| IBIS file stm32f373_378_383_lqfp64.ibs
[IBIS ver] 4.2
[File name] stm32f373_378_383_lqfp64.ibs
[File Rev] 1.0
[Date]  29-09-2025
[Source] Data Created at STMicroelectronics
[Notes]  File originated from ELDO simulations.
[Disclaimer]  This information is for modeling purpose only and is
   not guaranted. The information is subject to change without
   notice.
[Copyright] Copyright 2025 STMicroelectronics Inc.
|   Component stm32f373_378_383_lqfp64
[Component] stm32f373_378_383_lqfp64
[Manufacturer] STMicroelectronics
[Package]
| variable   typ   min   max
R_pkg  0  NA  NA
L_pkg  0  NA  NA
C_pkg  0  NA  NA
[Pin]   signal_name   model_name R_pin  L_pin C_pin
1 VBAT POWER 0.06898 4.22E-09 1.2E-13
2 PC13 io8p_sudq_tc_v33 0.063756122 3.67878E-09 9.34694E-14
3 PC14-OSC32IN io8p_sudq_tc_v33 0.059335918 3.22082E-09 7.10204E-14
4 PC15-OSC32OUT io8p_sudq_tc_v33 0.055719388 2.84612E-09 5.26531E-14
5 PF0/OSC_IN io8p_wsudqh_i2c_ft 0.052906531 2.55469E-09 3.83673E-14
6 PF1/OSC_OUT io8p_wsudqh_i2c_ft 0.050897347 2.34653E-09 2.81633E-14
7 NRST ioreset_tc_v33 0.049691837 2.22163E-09 2.20408E-14
8 PC0 io8p_sudq_ft 0.04929 2.18E-09 2E-14
9 PC1 io8p_sudq_ft 0.04929 2.18E-09 2E-14
10 PC2 io8p_sudq_ft 0.049691837 2.22163E-09 2.20408E-14
11 PC3 io8p_sudq_ft 0.050897347 2.34653E-09 2.81633E-14
12 VSSA/VREF- GND 0.052906531 2.55469E-09 3.83673E-14
13 VDDA POWER 0.055719388 2.84612E-09 5.26531E-14
14 PA0 io8p_sudq_ft 0.059335918 3.22082E-09 7.10204E-14
15 PA1 io8p_sudq_ft 0.063756122 3.67878E-09 9.34694E-14
16 PA2 io8p_sudq_ft 0.06898 4.22E-09 1.2E-13
17 VREF+ POWER 0.06898 4.22E-09 1.2E-13
18 PA3 io8p_sudq_ft 0.063756122 3.67878E-09 9.34694E-14
19 VDD POWER 0.059335918 3.22082E-09 7.10204E-14
20 PA4 io8p_sudq_ft 0.055719388 2.84612E-09 5.26531E-14
21 PA5 io8p_sudq_ft 0.052906531 2.55469E-09 3.83673E-14
22 PA6 io8p_sudq_ft 0.050897347 2.34653E-09 2.81633E-14
23 PA7 io8p_sudq_ft 0.049691837 2.22163E-09 2.20408E-14
24 PC4 io8p_sudq_ft 0.04929 2.18E-09 2E-14
25 PC5 io8p_sudq_ft 0.04929 2.18E-09 2E-14
26 PB0 io8p_sudq_ft 0.049691837 2.22163E-09 2.20408E-14
27 PB1 io8p_sudq_ft 0.050897347 2.34653E-09 2.81633E-14
28 PB2 io8p_sudq_ft 0.052906531 2.55469E-09 3.83673E-14
29 PE8 io8p_sudq_ft 0.055719388 2.84612E-09 5.26531E-14
30 PE9 io8p_sudq_ft 0.059335918 3.22082E-09 7.10204E-14
31 VSSSD/VREFSD- GND 0.063756122 3.67878E-09 9.34694E-14
32 VDDSD POWER 0.06898 4.22E-09 1.2E-13
33 VREFSD+ POWER 0.06898 4.22E-09 1.2E-13
34 PB14 io8p_sudq_ft 0.063756122 3.67878E-09 9.34694E-14
35 PB15 io8p_sudq_ft 0.059335918 3.22082E-09 7.10204E-14
36 PD8 io8p_sudq_ft 0.055719388 2.84612E-09 5.26531E-14
37 PC6 io8p_sudq_ft 0.052906531 2.55469E-09 3.83673E-14
38 PC7 io8p_sudq_ft 0.050897347 2.34653E-09 2.81633E-14
39 PC8 io8p_sudq_ft 0.049691837 2.22163E-09 2.20408E-14
40 PC9 io8p_sudq_ft 0.04929 2.18E-09 2E-14
41 PA8 io8p_sudq_ft 0.04929 2.18E-09 2E-14
42 PA9 io8p_wsudqh_i2c_ft 0.049691837 2.22163E-09 2.20408E-14
43 PA10 io8p_wsudqh_i2c_ft 0.050897347 2.34653E-09 2.81633E-14
44 PA11 io8usb_lv_ft 0.052906531 2.55469E-09 3.83673E-14
45 PA12 io8usb_lv_ft 0.055719388 2.84612E-09 5.26531E-14
46 PA13 io8p_sudq_ft 0.059335918 3.22082E-09 7.10204E-14
47 PF6 io8p_wsudqh_i2c_ft 0.063756122 3.67878E-09 9.34694E-14
48 PF7 io8p_wsudqh_i2c_ft 0.06898 4.22E-09 1.2E-13
49 PA14 io8p_wsudqh_i2c_ft 0.06898 4.22E-09 1.2E-13
50 PA15 io8p_wsudqh_i2c_ft 0.063756122 3.67878E-09 9.34694E-14
51 PC10 io8p_sudq_ft 0.059335918 3.22082E-09 7.10204E-14
52 PC11 io8p_sudq_ft 0.055719388 2.84612E-09 5.26531E-14
53 PC12 io8p_sudq_ft 0.052906531 2.55469E-09 3.83673E-14
54 PD2 io8p_sudq_ft 0.050897347 2.34653E-09 2.81633E-14
55 PB3 io8p_sudq_ft 0.049691837 2.22163E-09 2.20408E-14
56 PB4 io8p_sudq_ft 0.04929 2.18E-09 2E-14
57 PB5 io8p_sudq_ft 0.04929 2.18E-09 2E-14
58 PB6 io8p_wsudqh_i2c_ft 0.049691837 2.22163E-09 2.20408E-14
59 PB7 io8p_wsudqh_i2c_ft 0.050897347 2.34653E-09 2.81633E-14
60 BOOT0 vpp_test_hv 0.052906531 2.55469E-09 3.83673E-14
61 PB8 io8p_wsudqh_i2c_ft 0.055719388 2.84612E-09 5.26531E-14
62 PB9 io8p_wsudqh_i2c_ft 0.059335918 3.22082E-09 7.10204E-14
63 VSS GND 0.063756122 3.67878E-09 9.34694E-14
64 VDD POWER 0.06898 4.22E-09 1.2E-13
[Model Selector] io8p_sudq_ft
io8p01_sudq_ft_pd_lv  "SPEED01 2P0V, PD=40kOhm"
io8p01_sudq_ft_pu_lv  "SPEED01 2P0V, PU=40kOhm"
io8p01_sudq_ft_lv  "SPEED01 2P0V"
io8p10_sudq_ft_pd_lv  "SPEED10 2P0V, PD=40kOhm"
io8p10_sudq_ft_pu_lv  "SPEED10 2P0V, PU=40kOhm"
io8p10_sudq_ft_lv  "SPEED10 2P0V"
io8p11_sudq_ft_pd_lv  "SPEED11 2P0V, PD=40kOhm"
io8p11_sudq_ft_pu_lv  "SPEED11 2P0V, PU=40kOhm"
io8p11_sudq_ft_lv  "SPEED11 2P0V"
io8p01_sudq_ft_pd  "SPEED01, PD=40kOhm"
io8p01_sudq_ft_pu  "SPEED01, PU=40kOhm"
io8p01_sudq_ft  "SPEED01"
io8p10_sudq_ft_pd  "SPEED10, PD=40kOhm"
io8p10_sudq_ft_pu  "SPEED10, PU=40kOhm"
io8p10_sudq_ft  "SPEED10"
io8p11_sudq_ft_pd  "SPEED11, PD=40kOhm"
io8p11_sudq_ft_pu  "SPEED11, PU=40kOhm"
io8p11_sudq_ft  "SPEED11"
[Model Selector] io8p_sudq_tc_v33
io8p01_sudq_tc_v33_pd_lv  "SPEED01 2P0V, PD=40kOhm"
io8p01_sudq_tc_v33_pu_lv  "SPEED01 2P0V, PU=40kOhm"
io8p01_sudq_tc_v33_lv  "SPEED01 2P0V"
io8p10_sudq_tc_v33_pd_lv  "SPEED10 2P0V, PD=40kOhm"
io8p10_sudq_tc_v33_pu_lv  "SPEED10 2P0V, PU=40kOhm"
io8p10_sudq_tc_v33_lv  "SPEED10 2P0V"
io8p11_sudq_tc_v33_pd_lv  "SPEED11 2P0V, PD=40kOhm"
io8p11_sudq_tc_v33_pu_lv  "SPEED11 2P0V, PU=40kOhm"
io8p11_sudq_tc_v33_lv  "SPEED11 2P0V"
io8p01_sudq_tc_v33_pd  "SPEED01, PD=40kOhm"
io8p01_sudq_tc_v33_pu  "SPEED01, PU=40kOhm"
io8p01_sudq_tc_v33  "SPEED01"
io8p10_sudq_tc_v33_pd  "SPEED10, PD=40kOhm"
io8p10_sudq_tc_v33_pu  "SPEED10, PU=40kOhm"
io8p10_sudq_tc_v33  "SPEED10"
io8p11_sudq_tc_v33_pd  "SPEED11, PD=40kOhm"
io8p11_sudq_tc_v33_pu  "SPEED11, PU=40kOhm"
io8p11_sudq_tc_v33  "SPEED11"
[Model Selector] io8p_wsudqh_i2c_ft
io8p_wsudqh_i2c_ft_lv_pd  "General purpose IO with I2C capability on. 5V tolerant. 1.8V range with pull down"
io8p_wsudqh_i2c_ft_lv_pu  "General purpose IO with I2C capability on. 5V tolerant. 1.8V range with pull up"
io8p_wsudqh_i2c_ft_lv  "General purpose IO with I2C capability on. 5V tolerant. 1.8V range"
io8p_wsudqh_i2c_ft_pd  "General purpose IO with I2C capability on. 5V tolerant. 3.3V range with pull down"
io8p_wsudqh_i2c_ft_pu  "General purpose IO with I2C capability on. 5V tolerant. 3.3V range with pull up"
io8p_wsudqh_i2c_ft_i2c  "General purpose IO with I2C capability on. 5V tolerant. 3.3V range"
[Model Selector] io8usb_lv_ft
io8usb_dpdn_lv_ft_pd  "FS USB DP/DN IO + PD=40kOhm"
io8usb_dpdn_lv_ft_pu  "FS USB DP/DN IO + PU=40kOhm"
io8usb_dpdn_lv_ft  "FS USB DP/DN IO"
io8p01_lv_ft_pd_lv  "SPEED01 2P0V, PD=40kOhm"
io8p01_lv_ft_pu_lv  "SPEED01 2P0V, PU=40kOhm"
io8p01_lv_ft_lv  "SPEED01 2P0V"
io8p10_lv_ft_pd_lv  "SPEED10 2P0V, PD=40kOhm"
io8p10_lv_ft_pu_lv  "SPEED10 2P0V, PU=40kOhm"
io8p10_lv_ft_lv  "SPEED10 2P0V"
io8p11_lv_ft_pd_lv  "SPEED11 2P0V, PD=40kOhm"
io8p11_lv_ft_pu_lv  "SPEED11 2P0V, PU=40kOhm"
io8p11_lv_ft_lv  "SPEED11 2P0V"
io8p01_lv_ft_pd  "SPEED01, PD=40kOhm"
io8p01_lv_ft_pu  "SPEED01, PU=40kOhm"
io8p01_lv_ft  "SPEED01"
io8p10_lv_ft_pd  "SPEED10, PD=40kOhm"
io8p10_lv_ft_pu  "SPEED10, PU=40kOhm"
io8p10_lv_ft  "SPEED10"
io8p11_lv_ft_pd  "SPEED11, PD=40kOhm"
io8p11_lv_ft_pu  "SPEED11, PU=40kOhm"
io8p11_lv_ft  "SPEED11"
[Model Selector] ioreset_tc_v33
ioreset_tc_v33_pu_lv  "IORESET 2V + PU=40kOhm"
ioreset_tc_v33_nopu_lv  "IORESET 2V"
ioreset_tc_v33_pu  "IORESET + PU=40kOhm"
ioreset_tc_v33_nopu  "IORESET"
[Model Selector] vpp_test_hv
vpp_test_hv_3p3  "Input Buffer"
vpp_test_hv_2p4  "Input Buffer 2P0V"
| Models and submodels in the file (69): io8p01_sudq_ft_pd_lv (I/O), io8p01_sudq_ft_pu_lv (I/O), io8p01_sudq_ft_lv (I/O), io8p10_sudq_ft_pd_lv (I/O), io8p10_sudq_ft_pu_lv (I/O), io8p10_sudq_ft_lv (I/O), io8p11_sudq_ft_pd_lv (I/O), io8p11_sudq_ft_pu_lv (I/O), io8p11_sudq_ft_lv (I/O), io8p01_sudq_ft_pd (I/O), io8p01_sudq_ft_pu (I/O), io8p01_sudq_ft (I/O), io8p10_sudq_ft_pd (I/O), io8p10_sudq_ft_pu (I/O), io8p10_sudq_ft (I/O), io8p11_sudq_ft_pd (I/O), io8p11_sudq_ft_pu (I/O), io8p11_sudq_ft (I/O), io8p01_sudq_tc_v33_pd_lv (I/O), io8p01_sudq_tc_v33_pu_lv (I/O), io8p01_sudq_tc_v33_lv (I/O), io8p10_sudq_tc_v33_pd_lv (I/O), io8p10_sudq_tc_v33_pu_lv (I/O), io8p10_sudq_tc_v33_lv (I/O), io8p11_sudq_tc_v33_pd_lv (I/O), io8p11_sudq_tc_v33_pu_lv (I/O), io8p11_sudq_tc_v33_lv (I/O), io8p01_sudq_tc_v33_pd (I/O), io8p01_sudq_tc_v33_pu (I/O), io8p01_sudq_tc_v33 (I/O), io8p10_sudq_tc_v33_pd (I/O), io8p10_sudq_tc_v33_pu (I/O), io8p10_sudq_tc_v33 (I/O), io8p11_sudq_tc_v33_pd (I/O), io8p11_sudq_tc_v33_pu (I/O), io8p11_sudq_tc_v33 (I/O), io8p_wsudqh_i2c_ft_lv_pd (I/O), io8p_wsudqh_i2c_ft_lv_pu (I/O), io8p_wsudqh_i2c_ft_lv (I/O), io8p_wsudqh_i2c_ft_pd (I/O), io8p_wsudqh_i2c_ft_pu (I/O), io8p_wsudqh_i2c_ft_i2c (I/O), io8usb_dpdn_lv_ft_pd (I/O), io8usb_dpdn_lv_ft_pu (I/O), io8usb_dpdn_lv_ft (I/O), io8p01_lv_ft_pd_lv (I/O), io8p01_lv_ft_pu_lv (I/O), io8p01_lv_ft_lv (I/O), io8p10_lv_ft_pd_lv (I/O), io8p10_lv_ft_pu_lv (I/O), io8p10_lv_ft_lv (I/O), io8p11_lv_ft_pd_lv (I/O), io8p11_lv_ft_pu_lv (I/O), io8p11_lv_ft_lv (I/O), io8p01_lv_ft_pd (I/O), io8p01_lv_ft_pu (I/O), io8p01_lv_ft (I/O), io8p10_lv_ft_pd (I/O), io8p10_lv_ft_pu (I/O), io8p10_lv_ft (I/O), io8p11_lv_ft_pd (I/O), io8p11_lv_ft_pu (I/O), io8p11_lv_ft (I/O), ioreset_tc_v33_pu_lv (I/O_open_drain), ioreset_tc_v33_nopu_lv (I/O_open_drain), ioreset_tc_v33_pu (I/O_open_drain), ioreset_tc_v33_nopu (I/O_open_drain), vpp_test_hv_2p4 (Input), vpp_test_hv_3p3 (Input)
